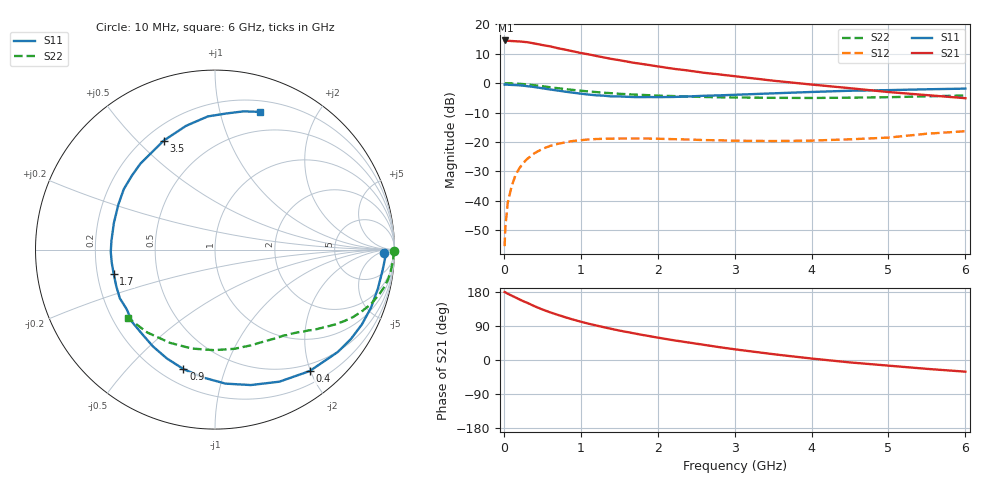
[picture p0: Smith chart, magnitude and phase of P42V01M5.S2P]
! SIEMENS Small Signal Semiconductors
! BFP182
! Si NPN RF Bipolar Junction Transistor in SOT143
! VCE = 2 V  IC = 1.5 mA
! Common Emitter S-Parameters:  March  1996
# GHz  S  MA  R  50
!  f  S11  S21  S12  S22
! GHz  MAG  ANG  MAG  ANG  MAG  ANG  MAG  ANG
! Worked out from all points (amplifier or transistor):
!   36 points, 10 MHz to 6 GHz, reference 50 ohm
!   highest |S21| = 14.5 dB at 20 MHz (marker M1)
!   |S21| within 3 dB of that: start of sweep to 774.4 MHz
!   unconditionally stable (mu >= 1): 2.378 GHz to end of sweep
!   at 250 MHz: K = 0.11, MSG = 20.6 dB, |S12| = -27.2 dB
!   at 1.4 GHz: K = 0.61, MSG = 13.5 dB, |S12| = -18.8 dB
!   at 6 GHz: K = 1.02, MAG = 4.8 dB, |S12| = -16.3 dB
!   S11 on the Smith chart (normalised r, x): 10 MHz: 30, -11; 400 MHz: 0.39, -1.99; 900 MHz: 0.29, -0.73; 1.7 GHz: 0.27, -0.11; 3.5 GHz: 0.27, +0.60; 6 GHz: 0.30, +1.33
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0.01  0.9434 -1.2  5.233 179.3  0.0017 82.6  0.9977 -0.5
0.02  0.9496 -2.6  5.312 178.6  0.0036 85.1  0.9919 -1.0
0.05  0.9412 -6.8  5.245 175.0  0.0092 87.4  0.9952 -2.6
0.1  0.9332 -13.5  5.195 170.1  0.0175 81.2  0.9896 -5.2
0.15  0.9274 -20.5  5.146 165.2  0.027 77.7  0.9848 -7.8
0.25  0.9064 -33.3  5.04 155.4  0.0436 70.2  0.9644 -12.7
0.3  0.8909 -39.8  4.971 151.3  0.0511 66.4  0.9498 -15.0
0.4  0.8579 -52.1  4.712 141.8  0.0647 59.3  0.9201 -19.3
0.5  0.8187 -64.0  4.445 133.4  0.0763 52.9  0.8867 -22.9
0.6  0.7806 -75.2  4.224 126.0  0.0857 47.2  0.8536 -26.3
0.7  0.749 -85.5  3.93 119.2  0.0928 42.2  0.8211 -29.1
0.9  0.6885 -104.8  3.471 106.7  0.1043 33.5  0.7666 -33.7
1.1  0.6409 -122.6  3.087 95.8  0.1105 26.7  0.7237 -37.6
1.4  0.5936 -146.0  2.581 82.1  0.1142 18.8  0.6742 -42.5
1.7  0.5803 -166.4  2.208 70.1  0.1148 13.5  0.6386 -46.9
1.9  0.5808 -178.7  2.019 62.7  0.1143 10.7  0.6228 -49.9
2.2  0.5826 165.2  1.759 52.3  0.1119 7.9  0.6032 -54.4
2.8  0.6201 138.2  1.408 33.9  0.1069 5.6  0.5751 -64.6
3.5  0.671 115.3  1.102 15.4  0.1038 6.9  0.5632 -79.0
4.5  0.7431 93.1  0.821 -6.4  0.1111 12.6  0.5663 -103.3
5.5  0.7866 78.3  0.626 -23.4  0.1383 16.2  0.5967 -129.4
6  0.8072 71.9  0.555 -30.8  0.1526 13.8  0.617 -142.1
